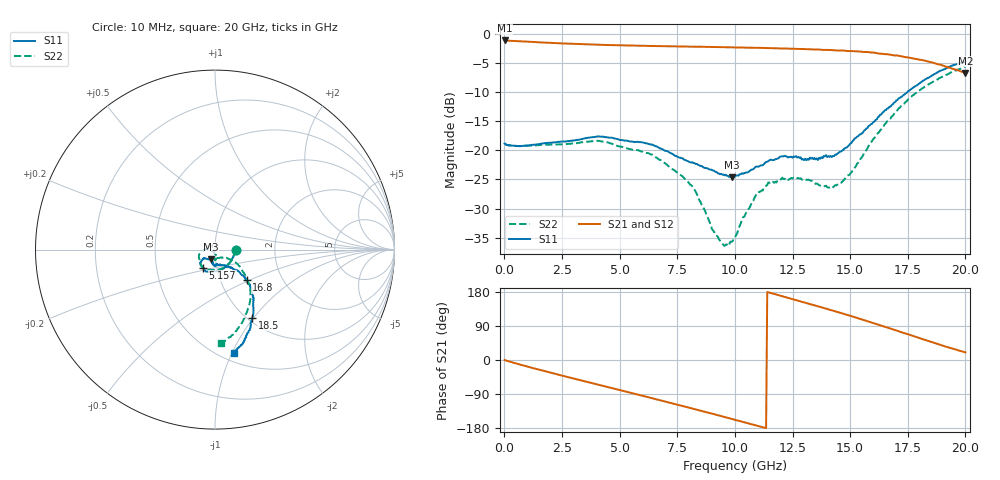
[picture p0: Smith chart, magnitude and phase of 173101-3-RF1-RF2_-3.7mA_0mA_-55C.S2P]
!  2-Port S-parameters saved by WinCal
! VAR MeasName=S-Parameters (CALIBRATED_DATA) read from VNA (N5242A)
! VAR MeasDate=2017-7-20 10:22:53
! VAR NAME=173101-3-RF1-RF2_-3.7mA_0mA_-55C
! VAR FILENAME=173101-3-RF1-RF2_-3.7mA_0mA_-55C.S2P
! VAR DATE=2017-7-20 10:22:53
! VAR PHYS_PORTS=1,2
# Hz S DB R 50
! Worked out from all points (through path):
!   401 points, 10 MHz to 20 GHz, reference 50 ohm
!   highest |S21| = -1.09 dB at 10 MHz (marker M1); lowest = -6.7 dB at 20 GHz (marker M2)
!   group delay of S21, straight-line fit = 46.5 ps
!   lowest |S11| = -24.6 dB at 9.855 GHz (marker M3), VSWR 1.12, Z = 47.5 - j5.16 ohm
!   |S11| at or under -10 dB: start of sweep to 17.48 GHz
!   |S22| runs from -36.5 to -5.6 dB; largest |S21 - S12| = 0.0072
!   S11 on the Smith chart (normalised r, x): 10 MHz: 1.26, -0.01; 5.157 GHz: 0.86, -0.18; 16.8 GHz: 1.33, -0.48; 18.5 GHz: 1.05, -0.98; 20 GHz: 0.58, -1.02
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1e7  -18.82 -2.2  -1.09 -0.0  -1.10 -0.1  -18.78 -2.0
1.50925e9  -18.91 -57.7  -1.42 -25.6  -1.43 -25.6  -19.10 -60.2
3.358325e9  -18.05 -99.9  -1.74 -54.3  -1.75 -54.3  -18.59 -108.8
4.10795e9  -17.61 -112.7  -1.84 -65.7  -1.85 -65.7  -18.37 -125.1
5.157425e9  -18.27 -123.8  -1.94 -81.7  -1.96 -81.7  -19.48 -141.7
6.70665e9  -19.54 -138.6  -2.06 -105.5  -2.06 -105.5  -21.56 -167.0
8.2059e9  -22.18 -142.4  -2.17 -128.9  -2.18 -128.9  -26.57 177.0
9.055475e9  -23.46 -126.2  -2.21 -142.3  -2.21 -142.4  -33.77 -160.8
9.455275e9  -24.18 -120.2  -2.25 -148.8  -2.25 -148.9  -35.96 -142.4
9.855075e9  -24.62 -113.0  -2.27 -155.3  -2.27 -155.4  -35.71 -113.5
1.0005e10  -24.41 -112.2  -2.29 -157.8  -2.30 -157.8  -34.91 -102.2
1.085458e10  -23.01 -101.7  -2.36 -171.6  -2.38 -171.7  -28.09 -79.8
1.145428e10  -21.81 -99.0  -2.41 178.6  -2.43 178.5  -25.51 -83.6
1.255372e10  -21.06 -88.3  -2.52 160.0  -2.54 160.0  -24.67 -89.8
1.335332e10  -21.26 -83.4  -2.64 146.2  -2.61 146.1  -25.24 -88.5
1.415292e10  -20.97 -71.3  -2.73 132.1  -2.75 131.9  -26.37 -78.2
1.465268e10  -20.04 -59.9  -2.81 123.1  -2.84 123.0  -25.38 -54.8
1.575212e10  -16.13 -45.1  -3.10 102.2  -3.11 102.1  -19.66 -32.1
1.670165e10  -12.52 -43.5  -3.51 83.8  -3.57 83.4  -14.65 -36.5
1.68016e10  -12.21 -44.3  -3.61 81.8  -3.61 82.0  -14.18 -38.0
1.850075e10  -7.29 -61.3  -4.82 48.0  -4.89 47.7  -8.42 -61.2
2e10  -4.67 -79.7  -6.67 20.3  -6.72 20.7  -5.62 -86.1
